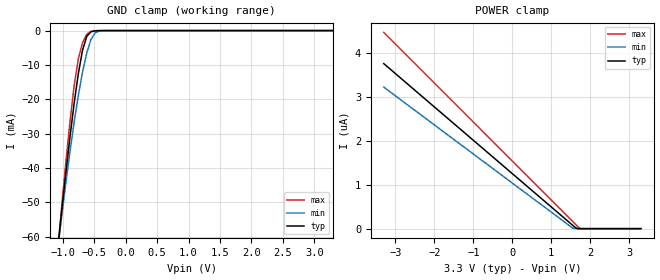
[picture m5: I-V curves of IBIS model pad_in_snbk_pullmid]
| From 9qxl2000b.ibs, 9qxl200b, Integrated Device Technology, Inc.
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|   Model pad_in_snbk_pullmid
[Model] pad_in_snbk_pullmid
Model_type Input
Vinl =   1.00V
Vinh =   2.00V
Polarity   Non-Inverting
C_comp   1.381pF   1.320pF   1.429pF
C_comp_pullup   85.534fF   84.274fF   87.188fF
[Temperature Range]   65.000   0.125k   -10.000
[Voltage Range]   3.300V   3.135V   3.465V
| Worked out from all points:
|   GND clamp passes 1 mA (typ) near -0.58 V on its own axis
[GND_clamp]
|Voltage   I(typ)   I(min)   I(max)
-3.3V     -515.8mA   -468.2mA   -566.4mA
-1.089V   -64.85mA   -64.84mA   -65.27mA
-1.022V   -53.13mA   -54.58mA   -51.76mA
-888mV    -31.15mA   -35.38mA   -26.75mA
-821mV    -21.27mA   -26.71mA   -16.12mA
-754mV    -12.57mA   -18.89mA   -8.247mA
-687mV    -5.728mA   -12.11mA   -3.539mA
-620mV    -1.705mA   -6.56mA    -1.08mA
-553mV    -365.9uA   -2.593mA   -222.6uA
-486mV    -74.23uA   -635.9uA   -35.42uA
-352mV    -3.869uA   -19.15uA   -2.226uA
3.3V      0A         0A         0A
[POWER_clamp]
|Voltage   I(typ)   I(min)   I(max)
-3.3V     3.768uA    3.232uA    4.481uA
1.558V    70.22nA    7.608nA    155.5nA
1.625V    19.23nA    0A         95.87nA
1.692V    0A         0A         36.21nA
1.759V    0A         0A         0A
3.3V      0A         0A         0A
